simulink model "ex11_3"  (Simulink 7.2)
settings: Solver=ode5  StartTime=0.0  StopTime=1  FixedStep=0.001  RelTol=1e-3

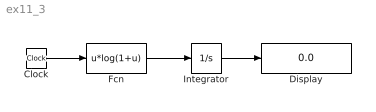
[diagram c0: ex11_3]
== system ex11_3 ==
  Clock : Clock
  Display : Display
  Fcn : Fcn  Expr=u*log(1+u)
  Integrator : Integrator
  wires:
  Clock/1 -> Fcn/1
  Fcn/1 -> Integrator/1
  Integrator/1 -> Display/1
